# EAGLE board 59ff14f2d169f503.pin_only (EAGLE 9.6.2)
REV: B

Size 71.12 x 71.12 mm. Coordinates in mm from the lower left corner, seen from the top.
Outline: 71.12,0 71.12,71.12 0,71.12 0,0 71.12,0
Copper layers (1*16): Top 0.035mm / dielectric 1.5mm / Bottom 0.035mm
Design rules "adafruit": minimum track width 8mil, minimum drill 15.5mil, track to track 8mil, track to pad 8mil, pad to pad 8mil, via to via 8mil, smd to smd 8mil, copper to edge 10mil, drill to drill 8mil, minimum pad ring 10mil, minimum via ring 8mil, stop-mask expansion 2mil, vias tented up to drill 20mil, thermal gap 10mil
Holes 2.8 mm at 17.78,2.54 35.56,2.54 53.34,2.54 53.34,68.58 35.56,68.58 17.78,68.58 8.89,26.67 8.89,44.45 35.56,26.67 35.56,44.45 62.23,26.67 62.23,44.45

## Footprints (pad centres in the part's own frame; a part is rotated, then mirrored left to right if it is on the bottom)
0805-NO = smd 1.24 x 1.5: 1 -0.95,0; 2 0.95,0
FIDUCIAL_1MM = smd 1 x 1: 1 0,0
1X03 = drill 1.016 pad 1.88: 1 0,0; 2 2.54,0; 3 5.08,0
WS2812B = smd 1.5 x 0.9: 1-VDD 2.45,-1.65; 2-DOUT 2.45,1.65; 3-GND -2.45,1.65; 4-DIN -2.45,-1.65
TESTPOINT_SMT = smd 4.7 x 3.4: P$1 0,0

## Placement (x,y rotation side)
C1  1.0uF  [0805-NO]  4.45,8.89 180 top
C2  1.0uF  [0805-NO]  4.45,17.78 180 top
C3  1.0uF  [0805-NO]  4.45,26.67 180 top
C4  1.0uF  [0805-NO]  4.45,35.56 180 top
C5  1.0uF  [0805-NO]  4.45,44.45 180 top
C6  1.0uF  [0805-NO]  4.45,53.34 180 top
C7  1.0uF  [0805-NO]  4.45,62.23 180 top
C9  1.0uF  [0805-NO]  13.34,8.89 180 top
C10  1.0uF  [0805-NO]  13.34,17.78 180 top
C11  1.0uF  [0805-NO]  13.34,26.67 180 top
C12  1.0uF  [0805-NO]  13.34,35.56 180 top
C13  1.0uF  [0805-NO]  13.34,44.45 180 top
C14  1.0uF  [0805-NO]  13.34,53.34 180 top
C15  1.0uF  [0805-NO]  13.34,62.23 180 top
C17  1.0uF  [0805-NO]  22.23,8.89 180 top
C18  1.0uF  [0805-NO]  22.23,17.78 180 top
C19  1.0uF  [0805-NO]  22.23,26.67 180 top
C20  1.0uF  [0805-NO]  22.23,35.56 180 top
C21  1.0uF  [0805-NO]  22.23,44.45 180 top
C22  1.0uF  [0805-NO]  22.23,53.34 180 top
C23  1.0uF  [0805-NO]  22.23,62.23 180 top
C25  1.0uF  [0805-NO]  31.11,8.89 180 top
C26  1.0uF  [0805-NO]  31.11,17.78 180 top
C27  1.0uF  [0805-NO]  31.11,26.67 180 top
C28  1.0uF  [0805-NO]  31.11,35.56 180 top
C29  1.0uF  [0805-NO]  31.11,44.45 180 top
C30  1.0uF  [0805-NO]  31.11,53.34 180 top
C31  1.0uF  [0805-NO]  31.11,62.23 180 top
C33  1.0uF  [0805-NO]  40.01,8.89 180 top
C34  1.0uF  [0805-NO]  40.01,17.78 180 top
C35  1.0uF  [0805-NO]  40.01,26.67 180 top
C36  1.0uF  [0805-NO]  40.01,35.56 180 top
C37  1.0uF  [0805-NO]  40.01,44.45 180 top
C38  1.0uF  [0805-NO]  40.01,53.34 180 top
C39  1.0uF  [0805-NO]  40.01,62.23 180 top
C41  1.0uF  [0805-NO]  48.9,8.89 180 top
C42  1.0uF  [0805-NO]  48.9,17.78 180 top
C43  1.0uF  [0805-NO]  48.9,26.67 180 top
C44  1.0uF  [0805-NO]  48.9,35.56 180 top
C45  1.0uF  [0805-NO]  48.9,44.45 180 top
C46  1.0uF  [0805-NO]  48.9,53.34 180 top
C47  1.0uF  [0805-NO]  48.9,62.23 180 top
C49  1.0uF  [0805-NO]  57.78,8.89 180 top
C50  1.0uF  [0805-NO]  57.78,17.78 180 top
C51  1.0uF  [0805-NO]  57.78,26.67 180 top
C52  1.0uF  [0805-NO]  57.78,35.56 180 top
C53  1.0uF  [0805-NO]  57.78,44.45 180 top
C54  1.0uF  [0805-NO]  57.78,53.34 180 top
C55  1.0uF  [0805-NO]  57.78,62.23 180 top
C57  1.0uF  [0805-NO]  66.67,8.89 180 top
C58  1.0uF  [0805-NO]  66.67,17.78 180 top
C59  1.0uF  [0805-NO]  66.67,26.67 180 top
C60  1.0uF  [0805-NO]  66.67,35.56 180 top
C61  1.0uF  [0805-NO]  66.67,44.45 180 top
C62  1.0uF  [0805-NO]  66.67,53.34 180 top
C63  1.0uF  [0805-NO]  66.67,62.23 180 top
FID1  FIDUCIAL_1MM  [FIDUCIAL_1MM]  17.4,5.46 90 top
FID2  FIDUCIAL_1MM  [FIDUCIAL_1MM]  62.23,8.51 90 top
FID3  FIDUCIAL_1MM  [FIDUCIAL_1MM]  9.27,62.23 90 top
JP1  [1X03]  8.89,1.91 90 top
JP2  [1X03]  62.23,68.96 270 top
LED1  WS2812B5050  [WS2812B]  4.45,4.45 90 top
LED2  WS2812B5050  [WS2812B]  4.45,13.34 90 top
LED3  WS2812B5050  [WS2812B]  4.45,22.23 90 top
LED4  WS2812B5050  [WS2812B]  4.45,31.11 90 top
LED5  WS2812B5050  [WS2812B]  4.45,40.01 90 top
LED6  WS2812B5050  [WS2812B]  4.45,48.9 90 top
LED7  WS2812B5050  [WS2812B]  4.45,57.78 90 top
LED8  WS2812B5050  [WS2812B]  4.45,66.67 90 top
LED9  WS2812B5050  [WS2812B]  13.34,4.45 90 top
LED10  WS2812B5050  [WS2812B]  13.34,13.34 90 top
LED11  WS2812B5050  [WS2812B]  13.34,22.23 90 top
LED12  WS2812B5050  [WS2812B]  13.34,31.11 90 top
LED13  WS2812B5050  [WS2812B]  13.34,40.01 90 top
LED14  WS2812B5050  [WS2812B]  13.34,48.9 90 top
LED15  WS2812B5050  [WS2812B]  13.34,57.78 90 top
LED16  WS2812B5050  [WS2812B]  13.34,66.67 90 top
LED17  WS2812B5050  [WS2812B]  22.23,4.45 90 top
LED18  WS2812B5050  [WS2812B]  22.23,13.34 90 top
LED19  WS2812B5050  [WS2812B]  22.23,22.23 90 top
LED20  WS2812B5050  [WS2812B]  22.23,31.11 90 top
LED21  WS2812B5050  [WS2812B]  22.23,40.01 90 top
LED22  WS2812B5050  [WS2812B]  22.23,48.9 90 top
LED23  WS2812B5050  [WS2812B]  22.23,57.78 90 top
LED24  WS2812B5050  [WS2812B]  22.23,66.67 90 top
LED25  WS2812B5050  [WS2812B]  31.11,4.45 90 top
LED26  WS2812B5050  [WS2812B]  31.11,13.34 90 top
LED27  WS2812B5050  [WS2812B]  31.11,22.23 90 top
LED28  WS2812B5050  [WS2812B]  31.11,31.11 90 top
LED29  WS2812B5050  [WS2812B]  31.11,40.01 90 top
LED30  WS2812B5050  [WS2812B]  31.11,48.9 90 top
LED31  WS2812B5050  [WS2812B]  31.11,57.78 90 top
LED32  WS2812B5050  [WS2812B]  31.11,66.67 90 top
LED33  WS2812B5050  [WS2812B]  40.01,4.45 90 top
LED34  WS2812B5050  [WS2812B]  40.01,13.34 90 top
LED35  WS2812B5050  [WS2812B]  40.01,22.23 90 top
LED36  WS2812B5050  [WS2812B]  40.01,31.11 90 top
LED37  WS2812B5050  [WS2812B]  40.01,40.01 90 top
LED38  WS2812B5050  [WS2812B]  40.01,48.9 90 top
LED39  WS2812B5050  [WS2812B]  40.01,57.78 90 top
LED40  WS2812B5050  [WS2812B]  40.01,66.67 90 top
LED41  WS2812B5050  [WS2812B]  48.9,4.45 90 top
LED42  WS2812B5050  [WS2812B]  48.9,13.34 90 top
LED43  WS2812B5050  [WS2812B]  48.9,22.23 90 top
LED44  WS2812B5050  [WS2812B]  48.9,31.11 90 top
LED45  WS2812B5050  [WS2812B]  48.9,40.01 90 top
LED46  WS2812B5050  [WS2812B]  48.9,48.9 90 top
LED47  WS2812B5050  [WS2812B]  48.9,57.78 90 top
LED48  WS2812B5050  [WS2812B]  48.9,66.67 90 top
LED49  WS2812B5050  [WS2812B]  57.78,4.45 90 top
LED50  WS2812B5050  [WS2812B]  57.78,13.34 90 top
LED51  WS2812B5050  [WS2812B]  57.78,22.23 90 top
LED52  WS2812B5050  [WS2812B]  57.78,31.11 90 top
LED53  WS2812B5050  [WS2812B]  57.78,40.01 90 top
LED54  WS2812B5050  [WS2812B]  57.78,48.9 90 top
LED55  WS2812B5050  [WS2812B]  57.78,57.78 90 top
LED56  WS2812B5050  [WS2812B]  57.78,66.67 90 top
LED57  WS2812B5050  [WS2812B]  66.67,4.45 90 top
LED58  WS2812B5050  [WS2812B]  66.67,13.34 90 top
LED59  WS2812B5050  [WS2812B]  66.67,22.23 90 top
LED60  WS2812B5050  [WS2812B]  66.67,31.11 90 top
LED61  WS2812B5050  [WS2812B]  66.67,40.01 90 top
LED62  WS2812B5050  [WS2812B]  66.67,48.9 90 top
LED63  WS2812B5050  [WS2812B]  66.67,57.78 90 top
LED64  WS2812B5050  [WS2812B]  66.67,66.67 90 top
R1  470 ohm  [0805-NO]  8.89,10.79 90 top
TP1  [TESTPOINT_SMT]  68.71,44.45 180 bottom
TP2  [TESTPOINT_SMT]  44.45,2.41 270 bottom
TP3  [TESTPOINT_SMT]  2.41,62.23 180 bottom
TP4  [TESTPOINT_SMT]  8.89,68.71 270 bottom
TP5  [TESTPOINT_SMT]  68.71,62.23 180 bottom
TP6  [TESTPOINT_SMT]  26.67,68.71 270 bottom
TP7  [TESTPOINT_SMT]  2.41,44.45 180 bottom
TP8  [TESTPOINT_SMT]  44.45,68.71 270 bottom
TP9  [TESTPOINT_SMT]  68.71,8.89 180 bottom
TP10  [TESTPOINT_SMT]  2.41,8.89 180 bottom
TP11  [TESTPOINT_SMT]  68.71,26.67 180 bottom
TP12  [TESTPOINT_SMT]  62.23,2.41 270 bottom
TP13  [TESTPOINT_SMT]  2.41,26.67 180 bottom
TP14  [TESTPOINT_SMT]  26.67,2.41 270 bottom
U$1  [ADAFRUIT_TEXT_30MM]  47.24,53.59 270 bottom
U$2  [PCBFEAT-REV-040]  62.1,35.43 90 top

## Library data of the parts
C1-C7 C9-C15 C17-C23 C25-C31 C33-C39 C41-C47 C49-C55 C57-C63 R1 TP1-TP14 = microbuilder
FID1-FID3 = microbuilder; BOM: EXCLUDE
JP1 JP2 U$1 = neomatrix-8x8
LED1-LED64 = microbuilder; ROT: 180
U$2 = microbuilder; REV: B

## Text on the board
tPlace: Only ONE Pin | 24 bit Color | Adafruit NeoPixel 8X8 | bLiNkY bLiNkY bLiNkY bLiNkY bLiNkY | 64 RGB LEDs
bPlace: DOUT | 5V | GND | Adafruit NeoPixel 8X8 | SKC6812 RGB LEDs | GND | 5V | DIN

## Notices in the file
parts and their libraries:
microbuilder: This work is placed in the public domain, and may be freely used for commercial and non-commercial work with the following conditions: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
